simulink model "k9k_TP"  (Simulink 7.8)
settings: Solver=ode3  StartTime=0.0  StopTime=10.0  RelTol=1e-3
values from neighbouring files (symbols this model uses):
  n = n+350    (= 1350)    [boucle.m]
undefined symbols (not defined in the file or in its folder): Z_pedal, Z_pilot, Z_pilotdemand, Z_prail, Z_timmain_nopil, Z_timmain_wpil
libraries: simulink x1

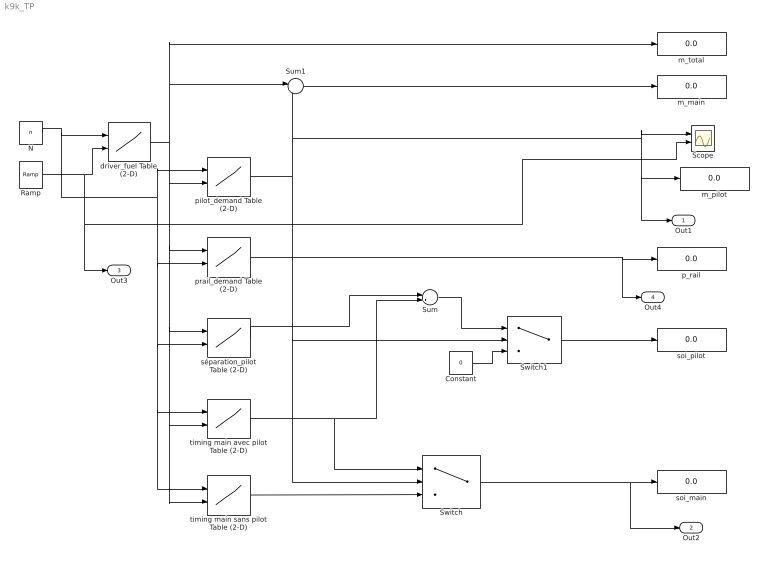
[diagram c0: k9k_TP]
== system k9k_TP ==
  Constant : Constant  Value=0
  N : Constant  Value=n
  Ramp : simulink/Sources/Ramp  slope=10  start=0  X0=0
  Scope : Scope  NumInputPorts=2
  Sum : Sum  Inputs=|++
  Sum1 : Sum  Inputs=|+-
  Switch : Switch  Threshold=0.2
  Switch1 : Switch  Criteria=u2 > Threshold  Threshold=0.2
  driver_fuel Table (2-D) : Lookup2D  RowIndex=Y_pedal  ColumnIndex=X_pedal  Table=Z_pedal
  m_main : Display
  m_pilot : Display
  m_total : Display
  p_rail : Display
  pilot_demand Table (2-D) : Lookup2D  RowIndex=Y_pilot_N  ColumnIndex=X_pilot_Q  Table=Z_pilot
  prail_demand Table (2-D) : Lookup2D  RowIndex=Y_prail  ColumnIndex=X_prail  Table=Z_prail
  soi_main : Display
  soi_pilot : Display
  séparation_pilot Table (2-D) : Lookup2D  RowIndex=Y_pilotdemand_n  ColumnIndex=X_pilotdemand_Q  Table=Z_pilotdemand
  timing main avec pilot Table (2-D) : Lookup2D  RowIndex=Y_timmain_wpil_N  ColumnIndex=X_timmain_wpil_Q  Table=Z_timmain_wpil
  timing main sans pilot Table (2-D) : Lookup2D  RowIndex=Y_timmain_nopil_N  ColumnIndex=X_timmain_nopil_Q  Table=Z_timmain_nopil
  Out1 : Outport
  Out2 : Outport  Port=2
  Out3 : Outport  Port=3
  Out4 : Outport  Port=4
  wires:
  prail_demand Table (2-D)/1 -> p_rail/1, Out4/1
  Switch/1 -> soi_main/1, Out2/1
  Switch1/1 -> soi_pilot/1
  Sum1/1 -> m_main/1
  Constant/1 -> Switch1/3
  Sum/1 -> Switch1/1
  séparation_pilot Table (2-D)/1 -> Sum/1
  timing main avec pilot Table (2-D)/1 -> Sum/2, Switch/1
  timing main sans pilot Table (2-D)/1 -> Switch/3
  pilot_demand Table (2-D)/1 -> Switch/2, Switch1/2, Sum1/2, Out1/1, m_pilot/1, Scope/1
  driver_fuel Table (2-D)/1 -> pilot_demand Table (2-D)/2, prail_demand Table (2-D)/1, séparation_pilot Table (2-D)/1, timing main avec pilot Table (2-D)/2, timing main sans pilot Table (2-D)/2, Sum1/1, m_total/1
  N/1 -> driver_fuel Table (2-D)/1, pilot_demand Table (2-D)/1, prail_demand Table (2-D)/2, séparation_pilot Table (2-D)/2, timing main avec pilot Table (2-D)/1, timing main sans pilot Table (2-D)/1
  Ramp/1 -> driver_fuel Table (2-D)/2, Out3/1, Scope/2
